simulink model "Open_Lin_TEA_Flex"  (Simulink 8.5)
settings: Solver=ode113  StartTime=0.0  StopTime=100000  RelTol=1e-3
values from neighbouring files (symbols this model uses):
  Kpqr = lqr(sys,Q0,R0)    [des.m]
  wo = 0.0011    [start.m]    (also in start1.m; start2.m; start3.m)
undefined symbols (not defined in the file or in its folder): Af, Bf, Cf, Df

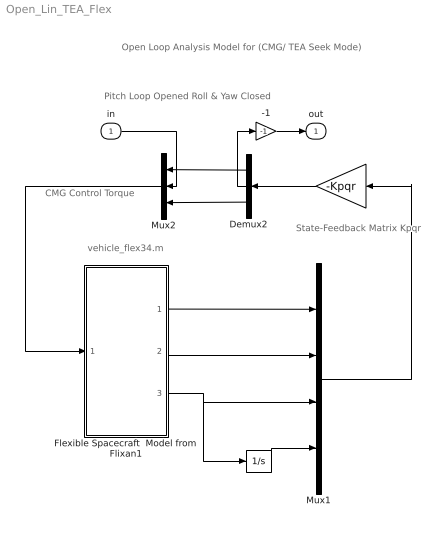
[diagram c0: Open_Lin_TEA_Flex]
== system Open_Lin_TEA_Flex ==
  note: Open Loop Analysis Model for (CMG/ TEA Seek Mode)
  note: CMG Control Torque
  note: State-Feedback Matrix Kpqr
  note: Pitch Loop Opened Roll & Yaw Closed
  note: vehicle_flex34.m
  in : Inport  PortDimensions=1
  " " : Gain  Gain=-Kpqr  Multiplication=Matrix(K*u)
  "  " : Integrator
  -1 : Gain  Gain=-1
  Demux2 : Demux  Outputs=3
  Flexible Spacecraft  Model from Flixan1 : Subsystem
  Mux1 : Mux  Inputs=[3, 3, 3, 3]
  Mux2 : Mux  Inputs=3
  out : Outport
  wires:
  Mux2/1 -> Flexible Spacecraft  Model from Flixan1/1(Tcmg)
  " "/1 -> Demux2/1
  -1/1 -> out/1
  Mux1/1 -> " "/1
  Flexible Spacecraft  Model from Flixan1/1(att-lv) -> Mux1/1
  Flexible Spacecraft  Model from Flixan1/2(w-lv) -> Mux1/2
  Flexible Spacecraft  Model from Flixan1/3("Hcmg ") -> "  "/1, Mux1/3
  "  "/1 -> Mux1/4
  Demux2/1 -> Mux2/1
  Demux2/3 -> Mux2/3
  in/1 -> Mux2/2
  Demux2/2 -> -1/1

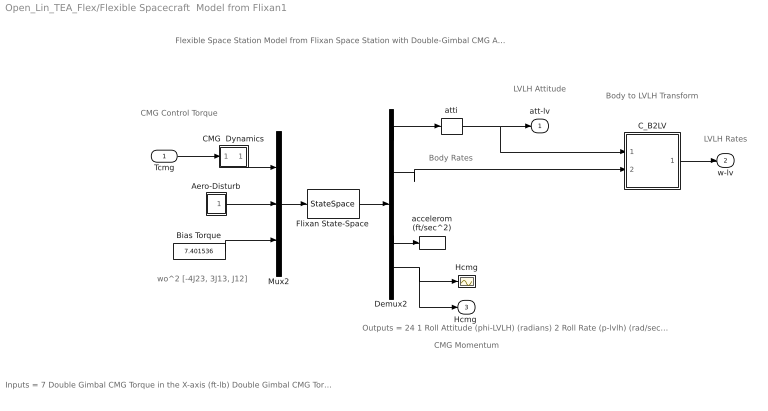
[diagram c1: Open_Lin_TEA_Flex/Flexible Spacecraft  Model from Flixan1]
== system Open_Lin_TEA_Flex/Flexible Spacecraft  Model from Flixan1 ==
  note: CMG Control Torque
  note: Body Rates
  note: LVLH Rates
  note: LVLH Attitude
  note: CMG Momentum
  note: wo^2 [-4J23, 3J13, J12]
  note: Body to LVLH Transform
  note: Outputs = 24 1 Roll Attitude (phi-LVLH) (radians) 2 Roll Rate (p-lvlh) (rad/sec) 3 Pitch Attitude (thet-LVLH) (radians) 4 Pitch Rate (q-lvlh) (rad/sec) 5 Yaw Attitude (psi-LVLH) (radians) 6 Yaw Rate (r-lvlh) (rad/sec) 7 Angle of attack, alfa, (radians) 8 Angle of sideslip, beta, (radian) 9 Change in Altitude, delta-h, (feet) 10 Forward Acceleration (V-dot) (ft/sec) 11 Cross Range Velocity (Vcr) (ft/sec) 12 Rate-Gyro # 1, Roll Rate (Body) (rad/sec) 13 Rate-Gyro # 2, Pitch Rate (Body) (rad/sec) 14 Rate-Gyro # 3, Yaw Rate (Body) (rad/sec) 15 Gyro # 4, Roll Attitude (Body) (radians) 16 Gyro # 5, Pitch Attitude (Body) (radians) 17 Gyro # 6, Yaw Attitude (Body) (radians) 18 Accelerom # 1, (along X), (ft/sec^2) Translat. Accelerat. 19 Accelerom # 2, (along Z), (ft/sec^2) Translat. Accelerat. 20 Accelerom # 3, (along X), (ft/sec^2) Translat. Accelerat. 21 Accelerom # 4, (along Z), (ft/sec^2) Translat. Accelerat. 22 Double Gimbal CMG Momentum Change in X-axis (ft-lb-sec) 23 Double Gimbal CMG Momentum Change in Y-axis (ft-lb-sec) 24 Double Gimbal CMG Momentum Change in Z-axis (ft-lb-sec)
  note: Flexible Space Station Model from Flixan Space Station with Double-Gimbal CMG Array (Flex)
  note: Inputs = 7 Double Gimbal CMG Torque in the X-axis (ft-lb) Double Gimbal CMG Torque in the Y-axis (ft-lb) Double Gimbal CMG Torque in the Z-axis (ft-lb) External Torque Input 1 (ft-lb), direct: External Torque Input 2 (ft-lb), direct: External Torque Input 3 (ft-lb), direct: Ext Torque Direct.=(0.197, -0.5964, -0.7782)
  Tcmg : Inport  PortDimensions=3
  Aero-Disturb : Subsystem
  Bias Torque : Constant  Value=7.401536
  CMG  Dynamics : Subsystem
  C_B2LV : Subsystem
  Demux2 : Demux  Outputs=[11, 3, 3, 4, 3]
  Flixan State-Space : StateSpace  A=Af  B=Bf  C=Cf  D=Df  X0=0
  Hcmg : Scope
  Mux2 : Mux  Inputs=[3, 3, 1]
  accelerom (ft/sec^2) : ToWorkspace  VariableName=accel  SampleTime=-1
  atti : Selector  InputPortWidth=11  Indices=[1 3 5]
  att-lv : Outport
  w-lv : Outport  Port=2
  "Hcmg " : Outport  Port=3
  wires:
  Aero-Disturb/1(Td) -> Mux2/2
  Tcmg/1 -> CMG  Dynamics/1(I)
  Demux2/2 -> C_B2LV/2(wb)
  Demux2/4 -> accelerom (ft/sec^2)/1
  atti/1 -> C_B2LV/1(atti), att-lv/1
  Demux2/1 -> atti/1
  Demux2/5 -> "Hcmg "/1, Hcmg/1
  Bias Torque/1 -> Mux2/3
  Flixan State-Space/1 -> Demux2/1
  Mux2/1 -> Flixan State-Space/1
  C_B2LV/1(wlv) -> w-lv/1
  CMG  Dynamics/1(O) -> Mux2/1

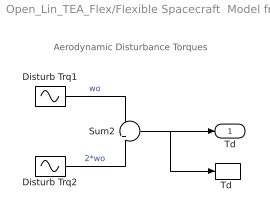
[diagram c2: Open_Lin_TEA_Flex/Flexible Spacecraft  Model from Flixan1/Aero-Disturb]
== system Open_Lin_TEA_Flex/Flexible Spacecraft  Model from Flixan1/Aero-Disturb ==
  note: Aerodynamic Disturbance Torques
  Disturb Trq1 : Sin  Amplitude=[1, 3, 1]  Bias="[1  8  1]"  Frequency=[wo, wo, wo]  SampleTime=0
  Disturb Trq2 : Sin  Amplitude=[1, 1, 1]*0.5  Frequency=[wo, wo, wo]*2  SampleTime=0
  Sum2 : Sum  Inputs=+|+
  "Td " : ToWorkspace  VariableName=Td  SampleTime=-1
  Td : Outport
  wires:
  Disturb Trq2/1 -> Sum2/2  "2*wo"
  Sum2/1 -> "Td "/1, Td/1
  Disturb Trq1/1 -> Sum2/1  "wo"

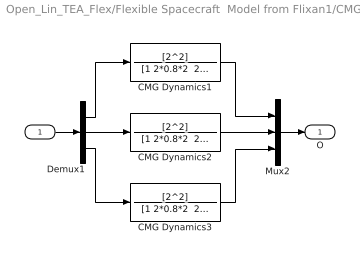
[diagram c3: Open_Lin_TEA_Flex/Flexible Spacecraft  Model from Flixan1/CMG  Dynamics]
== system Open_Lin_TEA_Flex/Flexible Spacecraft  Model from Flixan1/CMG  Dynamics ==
  I : Inport
  CMG Dynamics1 : TransferFcn  Numerator=[2^2]  Denominator="[1 2*0.8*2  2^2]"
  CMG Dynamics2 : TransferFcn  Numerator=[2^2]  Denominator="[1 2*0.8*2  2^2]"
  CMG Dynamics3 : TransferFcn  Numerator=[2^2]  Denominator="[1 2*0.8*2  2^2]"
  Demux1 : Demux  Outputs=3
  Mux2 : Mux  Inputs=3
  O : Outport
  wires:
  Mux2/1 -> O/1
  I/1 -> Demux1/1
  Demux1/3 -> CMG Dynamics3/1
  Demux1/1 -> CMG Dynamics1/1
  Demux1/2 -> CMG Dynamics2/1
  CMG Dynamics1/1 -> Mux2/1
  CMG Dynamics3/1 -> Mux2/3
  CMG Dynamics2/1 -> Mux2/2

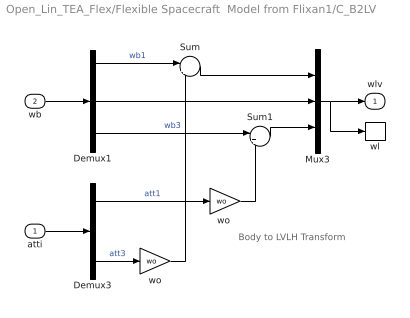
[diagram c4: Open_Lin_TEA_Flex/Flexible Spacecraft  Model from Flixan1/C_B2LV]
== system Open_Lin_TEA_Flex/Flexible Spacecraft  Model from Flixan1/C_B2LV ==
  note: Body to LVLH Transform
  atti : Inport  PortDimensions=3
  wb : Inport  Port=2  PortDimensions=3
  Demux1 : Demux  Outputs=3
  Demux3 : Demux  Outputs=3
  Mux3 : Mux  Inputs=3
  Sum : Sum  Inputs=|++
  Sum1 : Sum  Inputs=|+-
  wl : ToWorkspace  VariableName=wl  SampleTime=-1
  wo : Gain  Gain=wo
  "wo " : Gain  Gain=wo
  wlv : Outport
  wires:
  "wo "/1 -> Sum1/2
  Demux1/3 -> Sum1/1  "wb3"
  wo/1 -> Sum/2
  Demux1/2 -> Mux3/2
  Demux3/1 -> "wo "/1  "att1"
  Mux3/1 -> wl/1, wlv/1
  wb/1 -> Demux1/1
  atti/1 -> Demux3/1
  Sum1/1 -> Mux3/3
  Demux3/3 -> wo/1  "att3"
  Sum/1 -> Mux3/1
  Demux1/1 -> Sum/1  "wb1"
